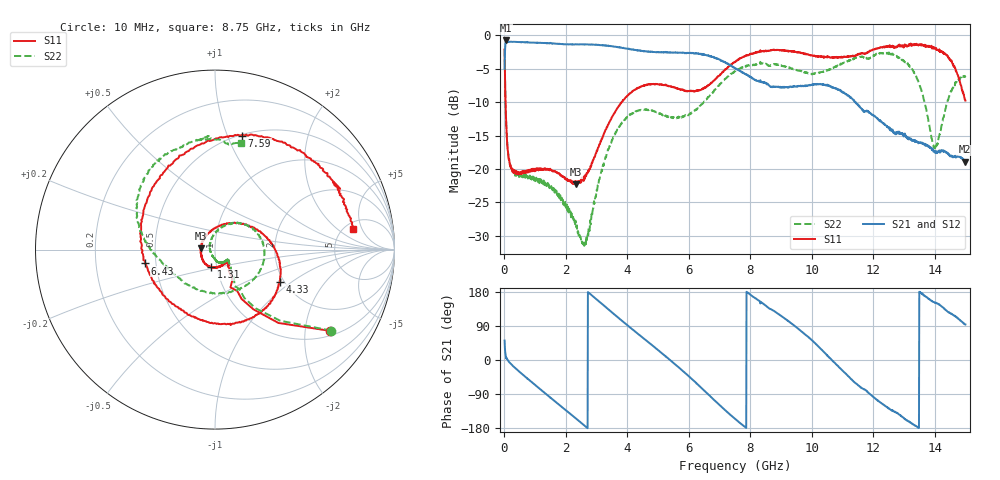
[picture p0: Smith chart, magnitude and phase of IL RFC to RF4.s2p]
!Agilent Technologies,N5230A,MY45001650,A.07.50.48
!Agilent N5230A: A.07.50.48
!Date: Wednesday, April 30, 2014 16:49:52
!Correction: S11(Full 2 Port(1,2))
!S21(Full 2 Port(1,2))
!S12(Full 2 Port(1,2))
!S22(Full 2 Port(1,2))
!S2P File: Measurements: S11, S21, S12, S22:
# Hz S  dB  R 50
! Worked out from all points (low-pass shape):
!   1500 points, 10 MHz to 15 GHz, reference 50 ohm
!   highest |S21| = -0.75 dB at 60 MHz (marker M1); lowest = -18.9 dB at 14.99 GHz (marker M2)
!   |S21| within 3 dB of the highest: 15.42 MHz to 7.038 GHz (7.023 GHz wide, 199 % of centre); 7.045078 GHz to 7.052541 GHz (7.462 MHz wide, 0.106 % of centre)
!   lowest |S11| = -22.3 dB at 2.34 GHz (marker M3), VSWR 1.17, Z = 42.9 + j0.571 ohm
!   |S11| at or under -10 dB: 39.52 MHz to 3.817 GHz (3.778 GHz wide, 196 % of centre)
!   |S22| runs from -31.6 to -2.1 dB; largest |S21 - S12| = 0.014
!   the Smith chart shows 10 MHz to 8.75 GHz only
!   S11 on the Smith chart (normalised r, x): 10 MHz: 1.15, -2.71; 1.31 GHz: 0.94, -0.18; 4.33 GHz: 1.90, -0.81; 6.43 GHz: 0.43, -0.08; 7.59 GHz: 0.51, +1.13; 8.75 GHz: 6.01, +3.42
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1e7  -2.12 -35.3  -5.00 51.3  -4.95 51.5  -2.07 -34.9
6e7  -12.87 -67.7  -0.75 4.2  -0.78 4.0  -12.78 -61.8
2.5e8  -20.11 -46.1  -0.97 -13.4  -0.96 -13.4  -20.01 -39.0
1.31e9  -20.08 -102.9  -1.13 -86.6  -1.12 -86.6  -22.24 -68.8
2.34e9  -22.27 175.1  -1.33 -154.9  -1.32 -155.0  -28.73 -116.6
2.51e9  -21.59 149.4  -1.33 -166.3  -1.35 -166.4  -30.85 -144.7
3.53e9  -12.01 29.2  -1.66 123.7  -1.63 123.8  -15.41 58.5
4.33e9  -7.91 -26.3  -2.28 70.2  -2.24 70.3  -11.27 3.1
5.01e9  -7.32 -64.3  -2.53 25.7  -2.55 25.7  -11.62 -50.9
5.72e9  -8.12 -106.3  -2.58 -22.9  -2.59 -22.6  -12.26 -117.5
6.43e9  -8.02 -168.8  -2.82 -75.2  -2.76 -75.1  -10.30 -167.4
7.51e9  -4.00 83.3  -4.94 -155.6  -4.95 -155.4  -5.34 140.4
7.59e9  -3.70 76.8  -5.12 -161.3  -5.18 -161.1  -5.19 136.6
8.75e9  -2.18 8.3  -7.74 130.6  -7.65 130.6  -4.30 76.3
1.001e10  -2.96 -63.5  -7.34 51.9  -7.43 51.9  -5.84 -14.9
1.067e10  -3.27 -116.4  -7.73 -1.5  -7.73 -1.6  -4.95 -68.9
1.128e10  -3.12 -179.7  -9.27 -50.6  -9.30 -50.1  -3.61 -108.5
1.251e10  -1.65 77.4  -13.75 -127.9  -13.79 -127.6  -2.54 -153.9
1.33e10  -1.36 42.5  -15.64 -169.5  -15.73 -168.2  -5.29 174.9
1.405e10  -1.90 9.5  -17.35 150.2  -17.40 150.3  -16.64 44.7
1.499e10  -9.60 -106.8  -18.93 93.8  -18.83 93.5  -6.21 -36.9
1.5e10  -9.76 -110.4  -18.90 93.7  -18.78 93.9  -6.08 -36.1
